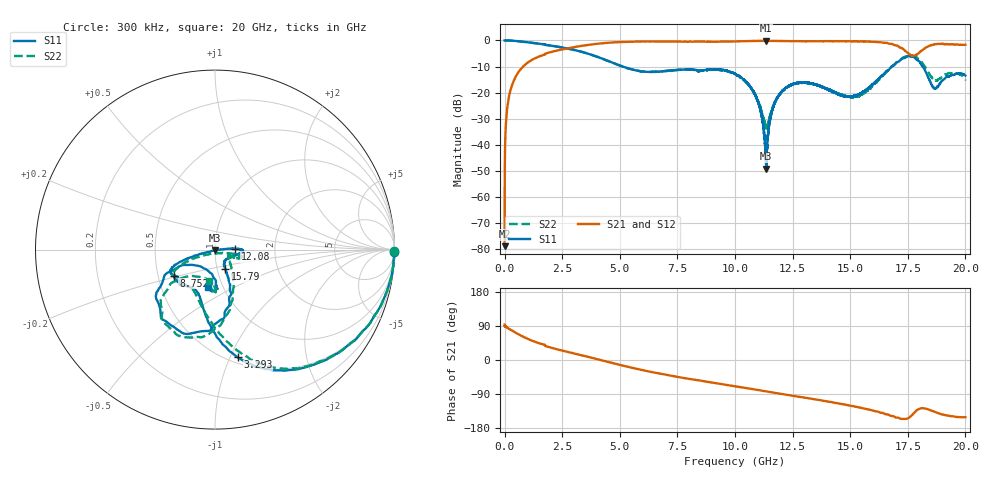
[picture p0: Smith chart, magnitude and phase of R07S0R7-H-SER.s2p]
!{R07S0R7}
!Johanson Technology Inc.
!www.johansontechnology.com
!Test Board Conditions:
!Substrate Type  RO4350B
!Substrate Thickness  10 mil
!Substrate Dk  3.66
!TL Type: GCPW
!TL Trace Width  21 mil
!TL Gap  20 mil
!Electrode orientation  Horizontal
!DUT TOPOLOGY	SERIES
!Mounting Pad LxW  16x21 mil
! Created Fri Feb  5 23:04:22 2021
# hz S ma R 50
! 2 Port Network Data from SP1.SP block
! freq  magS11  angS11  magS21  angS21  magS12  angS12  magS22  angS22
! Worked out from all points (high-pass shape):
!   20001 points, 300 kHz to 20 GHz, reference 50 ohm
!   highest |S21| = -0.14 dB at 11.33 GHz (marker M1); lowest = -79.0 dB at 300 kHz (marker M2)
!   |S21| within 3 dB of the highest: 2.659 GHz to 17.28 GHz (14.62 GHz wide, 147 % of centre); 18.22 GHz to end of sweep
!   lowest |S11| = -49.2 dB at 11.36 GHz (marker M3), VSWR 1.01, Z = 50.1 - j0.336 ohm
!   |S11| at or under -10 dB: 5.121849 GHz to 5.122796 GHz (946.4 kHz wide, 0.0185 % of centre); 5.124 GHz to 16.79 GHz (11.66 GHz wide, 106 % of centre); 18.14 GHz to end of sweep
!   |S22| runs from -33.9 to 0.0 dB; largest |S21 - S12| = 0.015
!   S11 on the Smith chart (normalised r, x): 300 kHz: open; 3.293 GHz: 0.56, -1.07; 8.752 GHz: 0.60, -0.19; 12.08 GHz: 1.25, +0.01; 15.79 GHz: 1.09, -0.24; 20 GHz: 0.85, -0.37
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300000  1 -0.6  0.0001126 93.2  0.0001997 76.7  0.9995 -0.6
1.293e8  0.9983 -5.0  0.05705 84.8  0.05698 84.9  0.9969 -5.0
4.853e8  0.9759 -17.7  0.2034 71.9  0.203 71.7  0.9776 -17.9
1.8503e9  0.8138 -54.6  0.5722 35.3  0.571 35.5  0.8134 -53.9
3.2933e9  0.6137 -78.0  0.7798 13.1  0.7799 13.1  0.6119 -74.5
3.3343e9  0.6077 -78.6  0.787 12.5  0.7856 12.5  0.6071 -75.1
6.6673e9  0.2519 -123.9  0.957 -35.2  0.9569 -35.2  0.2536 -126.5
8.7523e9  0.2721 -147.9  0.9473 -57.1  0.9485 -57.1  0.2699 -146.3
1.00003e10  0.2301 -159.3  0.9583 -69.1  0.9602 -69.2  0.2261 -155.1
1.09073e10  0.0835 -163.1  0.9787 -78.3  0.9796 -78.2  0.08459 -155.2
1.13303e10  0.006443 -121.4  0.984 -82.5  0.9809 -82.4  0.02243 -100.3
1.13593e10  0.00346 -75.8  0.9823 -82.8  0.9821 -82.8  0.02197 -87.7
1.16513e10  0.05121 1.7  0.9787 -85.9  0.9797 -86.0  0.05437 -22.0
1.20793e10  0.1105 2.4  0.974 -90.2  0.9763 -90.3  0.1085 -12.4
1.33343e10  0.1502 -6.6  0.966 -102.5  0.9681 -102.5  0.1492 -18.8
1.48363e10  0.08402 -40.4  0.9675 -118.4  0.9679 -118.4  0.08508 -22.7
1.57893e10  0.1227 -62.4  0.9495 -130.5  0.952 -130.5  0.1113 -41.5
1.66673e10  0.2713 -71.9  0.8693 -144.5  0.8728 -145.1  0.2737 -68.4
1.74643e10  0.4904 -107.2  0.5936 -155.1  0.5987 -154.9  0.5 -102.7
1.79283e10  0.4185 -142.1  0.5453 -131.3  0.5492 -131.9  0.4503 -130.5
1.86593e10  0.1213 -122.5  0.8424 -136.6  0.8419 -136.5  0.1738 -118.5
2e10  0.2116 -100.9  0.8295 -150.9  0.8272 -150.8  0.1793 -100.9
